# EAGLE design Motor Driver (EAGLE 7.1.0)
CNAME: Bristol Community College; CREVISION: v1r0; DESIGNER: J. Brian
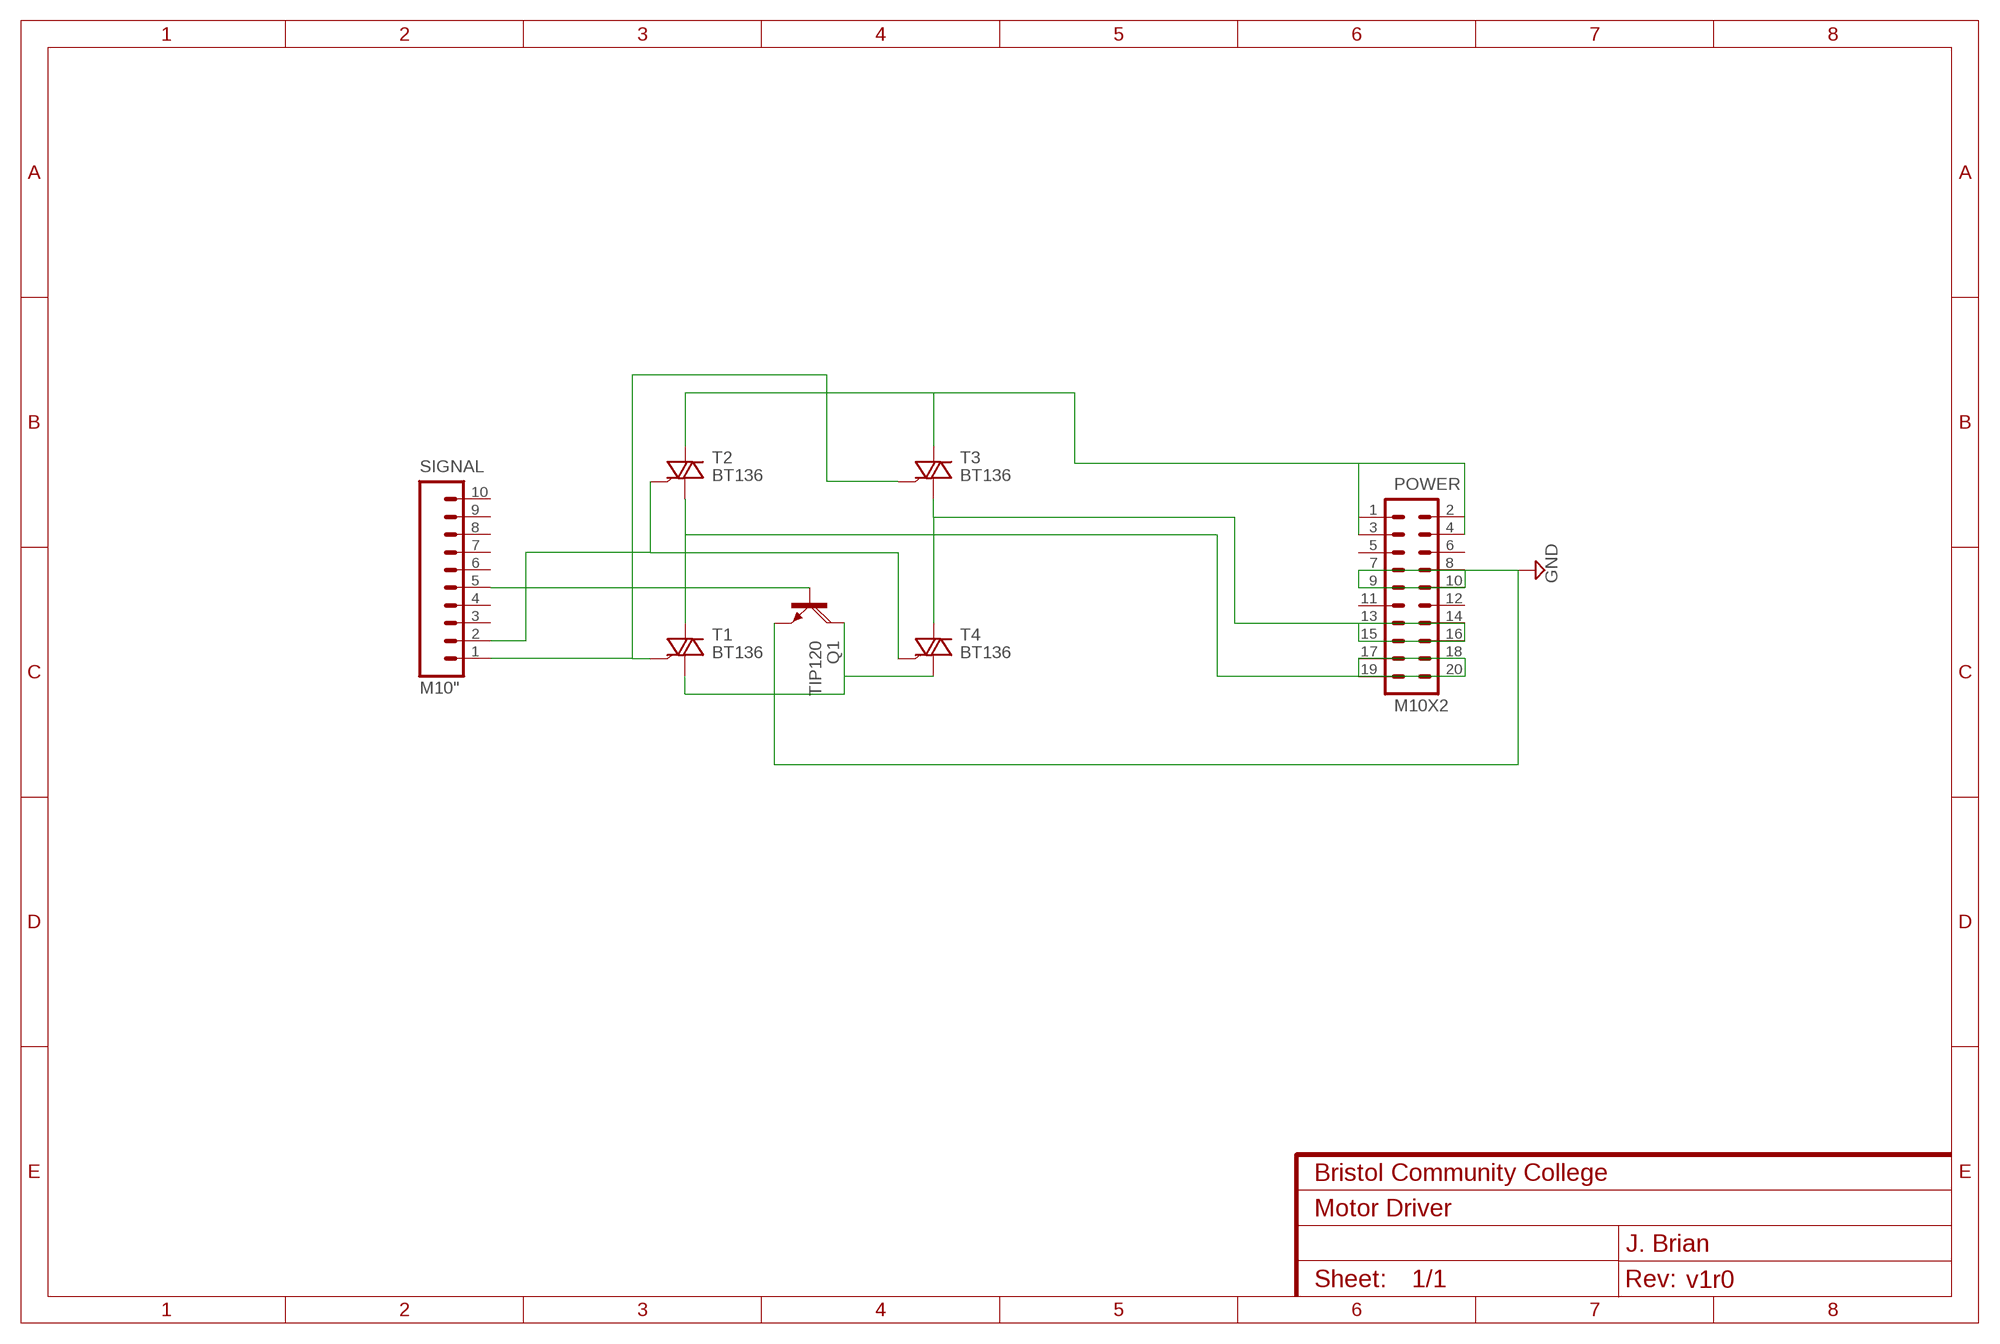
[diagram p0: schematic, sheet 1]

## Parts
POWER  M10X2  [2X10]
Q1  TIP120  [TO220AH]
SIGNAL  M10"  [1X10]
T1  BT136  [TO220AB]
T2  BT136  [TO220AB]
T3  BT136  [TO220AB]
T4  BT136  [TO220AB]

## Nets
GND: POWER.7 POWER.8 POWER.9 POWER.10 Q1.E
N$1: POWER.1 POWER.2 POWER.3 POWER.4 T2.2(A2) T3.2(A2)
N$2: POWER.13 POWER.14 POWER.15 POWER.16 T3.1(A1) T4.2(A2)
N$3: SIGNAL.2 T2.3(G) T4.3(G)
N$4: SIGNAL.1 T1.3(G) T3.3(G)
N$5: Q1.C T1.1(A1) T4.1(A1)
N$6: POWER.17 POWER.18 POWER.19 POWER.20 T1.2(A2) T2.1(A1)
N$11: Q1.B SIGNAL.5
Unconnected: POWER.5 POWER.6 POWER.11 POWER.12 SIGNAL.3 SIGNAL.4 SIGNAL.6 SIGNAL.7 SIGNAL.8 SIGNAL.9 SIGNAL.10

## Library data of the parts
POWER = SparkFun-Connectors:M10X2: This was SPECIALLY designed to be used with our Graphic LCD Backpack. Be sure you want to use this! It is not only staggered on each line of header holes, but IT IS ALSO offset of the center point of the top and bottom lines by 5 mil. This causes the headers to lock into place on the "standard"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
Q1 = transistor-power:TIP120: NPN DARLINGTON TRANSISTOR
SIGNAL = SparkFun-Connectors:M10: Header 10 Standard 10-pin 0.1" header. Use with straight break away headers (SKU : PRT-00116), right angle break away headers (PRT-00553), swiss pins (PRT-00743), machine pins (PRT-00117), and female headers (PRT-00115).
T1-T4 = triac:BT136: Triac BT136 series E sensitive gate Source: http://www.nxp.com/acrobat_download/datasheets/BT136_SERIES_E_2.pdf

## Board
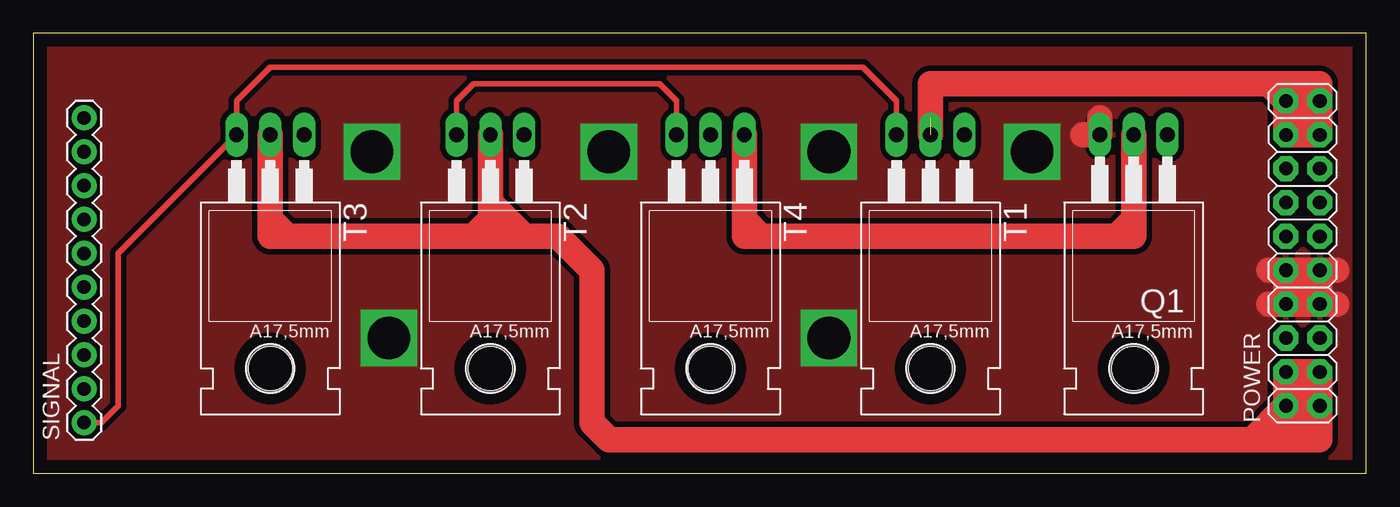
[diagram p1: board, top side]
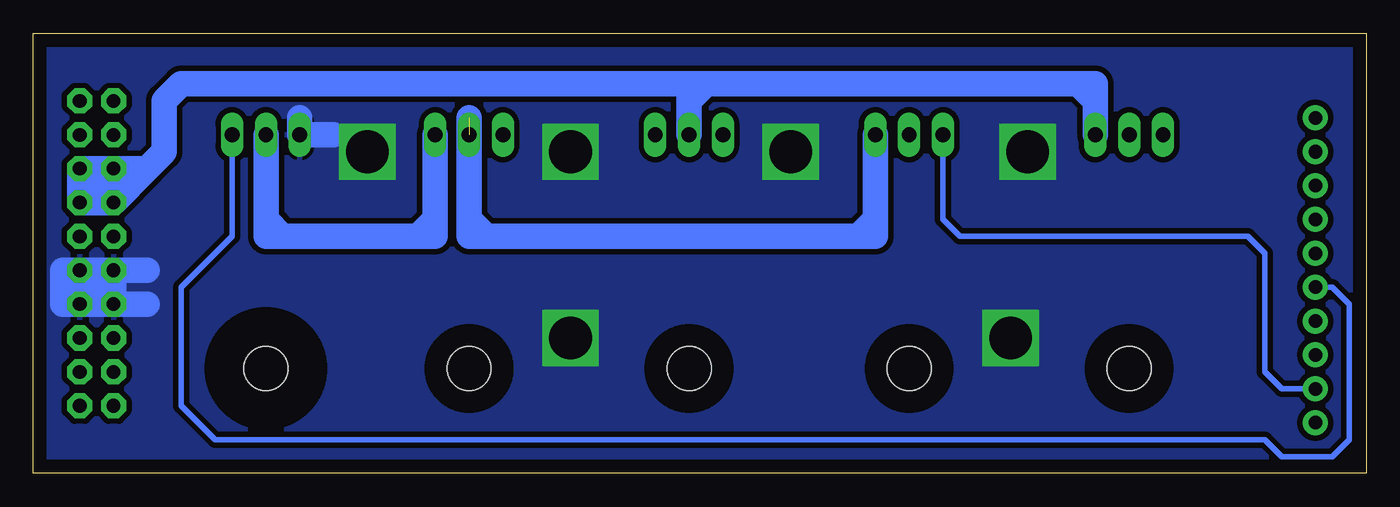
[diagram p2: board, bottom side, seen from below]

Size 100 x 33.01 mm. Coordinates in mm from the lower left corner, seen from the top.
Outline: 0,0 100,0 100,33.01 0,33.01 0,0
Copper layers (1*16): Top 0.035mm / dielectric 1.5mm / Bottom 0.035mm
Design rules "default": minimum track width 10mil, minimum drill 24mil, track to track 8mil, track to pad 8mil, pad to pad 8mil, via to via 8mil, smd to smd 8mil, copper to edge 40mil, drill to drill 8mil, minimum pad ring 10mil, minimum via ring 8mil, stop-mask expansion 4mil, vias tented up to drill 0mil, thermal gap 10mil

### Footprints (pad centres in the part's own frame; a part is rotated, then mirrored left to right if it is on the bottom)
2X10 = drill 1.016 pad 1.88 octagon: 1 -11.43,-1.27; 2 -11.43,1.27; 3 -8.89,-1.27; 4 -8.89,1.27; 5 -6.35,-1.27; 6 -6.35,1.27; 7 -3.81,-1.27; 8 -3.81,1.27; 9 -1.27,-1.27; 10 -1.27,1.27; 11 1.27,-1.27; 12 1.27,1.27; 13 3.81,-1.27; 14 3.81,1.27; 15 6.35,-1.27; 16 6.35,1.27; 17 8.89,-1.27; 18 8.89,1.27; 19 11.43,-1.27; 20 11.43,1.27
TO220AH = drill 1.118 long: B -2.54,-6.35; C 0,-6.35; E 2.54,-6.35 | hole 3.302: 0,11.176
1X10 = drill 1.016 pad 1.88: 1 0,0; 2 2.54,0; 3 5.08,0; 4 7.62,0; 5 10.16,0; 6 12.7,0; 7 15.24,0; 8 17.78,0; 9 20.32,0; 10 22.86,0
TO220AB = drill 1.118 long: 1 -2.54,-6.35; 2 0,-6.35; 3 2.54,-6.35 | hole 3.302: 0,11.176

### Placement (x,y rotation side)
POWER  95.25,16.51 90 top
Q1  82.55,19.05 180 top
SIGNAL  3.81,3.81 90 top
T1  67.31,19.05 180 top
T2  34.29,19.05 180 top
T3  17.78,19.05 180 top
T4  50.8,19.05 180 top

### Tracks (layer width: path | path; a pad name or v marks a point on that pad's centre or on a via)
GND  (via drill 3.2)
  Top 1.93: 80.01,26.67 Q1.E 78.74,25.4 | POWER.10 92.71,15.24 | POWER.10 POWER.9 | 97.79,15.24 POWER.9 | POWER.9 POWER.7 | POWER.7 97.79,12.7 | POWER.7 POWER.8 | 92.71,12.7 POWER.8 | POWER.8 POWER.10 | POWER.10 95.25,13.97
  Bottom 1.93: 77.47,25.4 Q1.E 80.01,26.67 | 91.44,15.24 POWER.10 | POWER.9 97.79,15.24 97.79,12.7 POWER.7 | POWER.7 POWER.8 | 91.44,12.7 POWER.8 | POWER.8 POWER.10 | POWER.10 POWER.9 | POWER.9 POWER.7 | POWER.7 95.25,13.97
  other vias: 25.4,24.13 43.18,24.13 59.69,24.13 26.67,10.16 59.69,10.16 74.93,24.13
  pour Bottom (isolate 0.406): 0,33.02 0,0 100.33,0 100.33,33.02
  pour Top (isolate 0.406): 0,33.02 0,0 100.33,0 100.33,33.02
N$1
  Top 1.93: T3.2 17.78,19.05 | 17.78,19.05 17.78,17.78 19.05,17.78 | 33.02,17.78 34.29,19.05 T2.2 34.29,20.32 36.83,17.78 | 36.83,17.78 33.02,17.78 | 33.02,17.78 19.05,17.78 | 19.05,17.78 17.78,19.05 | 36.83,17.78 39.37,17.78 41.91,15.24 41.91,3.81 43.18,2.54 91.44,2.54 | 91.44,2.54 POWER.2 | POWER.2 POWER.4 POWER.3 POWER.1 | POWER.1 POWER.2 | POWER.2 95.25,6.35 | POWER.1 96.52,2.54 91.44,2.54
N$2
  Bottom 1.93: T3.1 20.32,27.94 | 20.32,27.94 21.59,29.21 | 21.59,29.21 49.53,29.21 | 49.53,29.21 50.8,27.94 T4.2 50.8,29.21 | 50.8,29.21 49.53,29.21 | 21.59,29.21 20.32,29.21 20.32,27.94 | 50.8,29.21 88.9,29.21 90.17,27.94 90.17,24.13 91.44,22.86 | 91.44,22.86 POWER.16 | POWER.16 95.25,22.86 | 95.25,22.86 POWER.15 POWER.13 POWER.14 | POWER.14 POWER.16 | POWER.16 95.25,21.59 | 95.25,22.86 95.25,21.59 | 95.25,21.59 POWER.14 | POWER.14 91.44,22.86
N$3
  Top 0.406: T2.3 31.75,27.94 33.02,29.21 46.99,29.21 48.26,27.94 T4.3
  Bottom 0.406: SIGNAL.2 6.35,6.35 7.62,7.62 7.62,16.51 8.89,17.78 30.48,17.78 31.75,19.05 T2.3
N$4
  Top 0.406: SIGNAL.1 5.08,3.81 6.35,5.08 6.35,16.51 T3.3 15.24,27.94 17.78,30.48 62.23,30.48 64.77,27.94 T1.3
N$5
  Top 1.93: T4.1 53.34,19.05 | 53.34,19.05 54.61,17.78 | 54.61,17.78 81.28,17.78 | 81.28,17.78 82.55,19.05 Q1.C 82.55,17.78 81.28,17.78 | 54.61,17.78 53.34,17.78 53.34,19.05
  Bottom 1.93: T1.1 69.85,19.05 | 69.85,19.05 69.85,17.78 71.12,17.78 | 81.28,17.78 82.55,19.05 Q1.C 82.55,17.78 81.28,17.78 | 81.28,17.78 71.12,17.78 | 71.12,17.78 69.85,19.05
N$6  (1 unrouted)
  Top 1.93: T1.2 67.31,29.21 92.71,29.21 | 92.71,29.21 POWER.20 | POWER.20 POWER.18 POWER.17 POWER.19 | POWER.19 POWER.20 | POWER.20 95.25,26.67 POWER.19 | POWER.19 96.52,29.21 92.71,29.21
  Bottom 1.93: T2.1 36.83,19.05 | 36.83,19.05 38.1,17.78 | 38.1,17.78 66.04,17.78 | 66.04,17.78 67.31,19.05 | 67.31,19.05 67.31,26.67 | 67.31,19.05 67.31,17.78 66.04,17.78 | 38.1,17.78 36.83,17.78 36.83,19.05
N$7
  Top 1.93: 93.98,3.81 95.25,3.81
N$11
  Bottom 0.406: SIGNAL.5 2.54,13.97 1.27,12.7 1.27,2.54 2.54,1.27 6.35,1.27 7.62,2.54 86.36,2.54 88.9,5.08 88.9,13.97 85.09,17.78 Q1.B

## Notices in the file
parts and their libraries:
SparkFun-Aesthetics: Licensing: Creative Commons ShareAlike 4.0 International - https://creativecommons.org/licenses/by-sa/4.0
